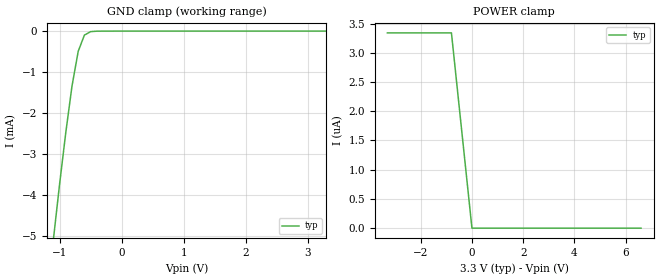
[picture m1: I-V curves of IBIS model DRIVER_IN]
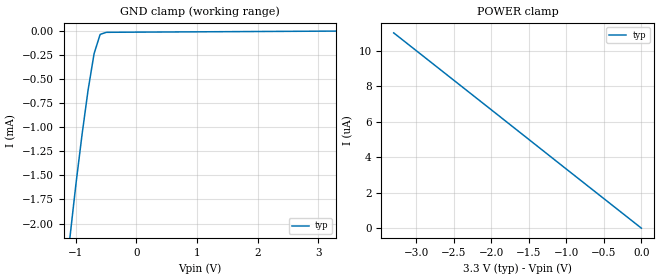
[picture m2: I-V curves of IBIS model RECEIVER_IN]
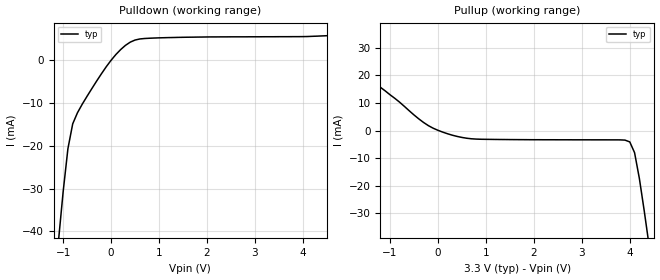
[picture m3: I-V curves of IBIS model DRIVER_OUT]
|   Texas Instruments Incorporated
|   Data Transmissions Products
|   IBIS Model for SN65LVDS179
|   8D SOIC Package
[IBIS Ver]   2.1
[Comment char]   |_char
[File name]   lvds179.ibs
[File Rev]   2.1
[Date]   03/24/2009
[Source]   File originated at Texas Instruments Incorporated.
   Data Transmission Products Group.
[Notes]   Revision History:
   Rev 2.0: 11/05/1998
   - Initial version
   Rev 2.1: 03/24/2009
   - Added Y and Z pins to [Diff pin] list
   - removed warning related to DRIVER_IN powerclamp
[Disclaimer]
(C) Copyright Texas Instruments Incorporated 1998
   All rights reserved
  Texas Instruments Incorporated hereby grants the user of this IBIS
model a non-exclusive, nontransferable license to use this IBIS model
under the following terms.  Before using this IBIS model, the user
should read this license.  If the user does not accept these terms,
the IBIS model should be returned to Texas Instruments within 30 days.
  The user is granted this license only to use the IBIS model and
is not granted rights to sell, load, rent, lease or license the IBIS
model in whole or in part, or in modified form to anyone other than
user.  User may modify the IBIS model to suit its specific applications
but rights to derivative works and such modifications shall belong to
Texas Instruments.
  This IBIS model is provided on an "AS IS" basis and Texas Instruments
makes absolutely no warranty with respect to the information contained
herein.  TEXAS INSTRUMENTS DISCLAIMS AND CUSTOMER WAIVES ALL WARRANTIES,
EXPRESS OR IMPLIED, INCLUDING WARRANTIES OF MERCHANTABILITY OR FITNESS
FOR A PARTICULAR PURPOSE. The entire risk as to quality and performance
is with the Customer. ACCORDINGLY, IN NO EVENT SHALL THE COMPANY BE LIABLE
FOR ANY DAMAGES, WHETHER IN CONTRACT OR TORT,INCLUDING ANY LOST PROFITS
OR OTHER INCIDENTAL, CONSEQUENTIAL, EXEMPLARY, OR PUNITIVE DAMAGES ARISING
OUT OF THE USE OR APPLICATION OF THE IBIS model provided in this package.
Further, Texas Instruments reserves the right to discontinue or make changes
without notice to any product herein to improve reliability, function, or
design. Texas Instruments does not convey any license under patent rights
or any other intellectual property rights, including those of third parties.
Contact Texas Instruments at ATTN:DATA TRANSMISSIONS
Thomas Fisher 8505 Forest Lane, M/S 8710, Dallas, TX 75243-4136
[Copyright]   Copyright 1998, Texas Instruments, All Rights Reserved
[Component]   LVDS179D
[Manufacturer]  Texas Instruments Incorporated
[Package]
|   typ   min   max
R_pkg   0.036   0.033   0.039
L_pkg   3.340nH   2.445nH   4.233nH
C_pkg   0.470pF   0.308pF   0.631pF
[Pin]   signal_name   model_name   R_pin   L_pin   C_pin
1   VCC   POWER   0.034   4.233n   0.630p
2   R   RECEIVER_OUT   0.038   2.445n   0.309p
3   D   DRIVER_IN   0.039   2.448n   0.309p
4   GND   GND   0.033   4.231n   0.631p
5   Y   DRIVER_OUT   0.033   4.230n   0.630p
6   Z   DRIVER_OUT   0.039   2.450n   0.308p
7   B   RECEIVER_IN   0.039   2.448n   0.309p
8   A   RECEIVER_IN   0.033   4.231n   0.630p
[Diff_pin]   inv_pin   vdiff   tdelay_typ   tdelay_min   tdelay_max
| The 'A' pin is Diff_pin and the 'B' pin is the inv_pin
8   7   0.100   0 0 0
5   6   0.300   0 0 0
| Models and submodels in the file (4): DRIVER_IN (Input), RECEIVER_IN (Input), DRIVER_OUT (Output), RECEIVER_OUT (Output)
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|   Driver Input MODEL
[Model]   DRIVER_IN
Model_type   Input
|Signals   D
Vinh = 2.0
Vinl = 0.8
|   typ   min   max
C_comp   1.0pF   NA   NA
|   typ   min   max
[Temperature Range]   25.0   NA   NA
[Voltage range]   3.3V   3.0V   3.6V
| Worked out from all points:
|   GND clamp passes 1 mA (typ) near -0.76 V on its own axis
[GND_clamp]
|   Voltage   I(typ)   I(min)   I(max)
-3.3V     -43.1mA    NA         NA
-1.1V     -5.08mA    NA         NA
-1V       -3.73mA    NA         NA
-900mV    -2.47mA    NA         NA
-800mV    -1.34mA    NA         NA
-700mV    -493uA     NA         NA
-600mV    -98.5uA    NA         NA
-500mV    -13.3uA    NA         NA
3.3V      3.34pA     NA         NA
[Power_clamp]
| Note that the[POWER_clamp]voltage table is referenced to Vcc
| and is calculated using Vtable=Vcc - Vmeasured.
|   Voltage   I(typ)   I(min)   I(max)
-3.3V     3.34uA     NA         NA
-2.7V     3.34uA     NA         NA
-2V       3.34uA     NA         NA
-800mV    3.34uA     NA         NA
0V        0A         NA         NA
6.6V      0A         NA         NA
|   Receiver Input MODEL
[Model]   RECEIVER_IN
Model_type   Input
|Signals   A,B
Vinh = 2.0
Vinl = 0.8
|   typ   min   max
C_comp   1.0pF   NA   NA
|   typ   min   max
[Temperature Range]   25.0   NA   NA
[Voltage range]   3.3V   3.0V   3.6V
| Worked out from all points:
|   GND clamp passes 1 mA (typ) near -0.88 V on its own axis
[GND_clamp]
|   Voltage   I(typ)   I(min)   I(max)
-3.3V     -22.5mA    NA         NA
-1.1V     -2.15mA    NA         NA
-1V       -1.59mA    NA         NA
-900mV    -1.08mA    NA         NA
-800mV    -616uA     NA         NA
-700mV    -234uA     NA         NA
-600mV    -34.5uA    NA         NA
-500mV    -13.2uA    NA         NA
-400mV    -12.3uA    NA         NA
3.3V      444pA      NA         NA
[Power_clamp]
| Note that the[POWER_clamp]voltage table is referenced to Vcc
| and is calculated using Vtable=Vcc - Vmeasured.
|   Voltage   I(typ)   I(min)   I(max)
-3.3V     11uA       NA         NA
-2V       6.67uA     NA         NA
-1V       3.33uA     NA         NA
0V        0A         NA         NA
|   Driver Output  MODEL
[Model]   DRIVER_OUT
Model_type   Output
| Signals   Y,Z
Vmeas = 1.2V   |Reference voltage for timing measurements
Cref = 5pF   |Timing specification test load capacitance value
Rref = 50   |Note: 50 Ohm load; single ended configuration
Vref = 1.18V   |Timing specification test load voltage
| variable   typ   min   max
C_comp   1.0pF   NA   NA
|   typ   min   max
[Temperature Range]   25.0   NA   NA
[Voltage range]   3.3V   3.0V   3.6V
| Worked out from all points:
|   slope of the pulldown table from 0 to 0.495 V, typ, clamps not added: 105 ohm
|   slope of the pullup table from 0 to 0.495 V, typ, clamps not added: 192 ohm
[Pulldown]
|   Voltage   I(typ)   I(min)   I(max)
-3.3V     -348mA     NA         NA
-1.1V     -42.6mA    NA         NA
-1V       -30.8mA    NA         NA
-900mV    -20.7mA    NA         NA
-800mV    -14.9mA    NA         NA
-600mV    -10.3mA    NA         NA
-100mV    -1.58mA    NA         NA
200mV     2.42mA     NA         NA
500mV     4.64mA     NA         NA
1.4V      5.26mA     NA         NA
4.1V      5.46mA     NA         NA
6.6V      7.11mA     NA         NA
[Pullup]
|   Voltage   I(typ)   I(min)   I(max)
| Note that the[Pullup]voltage table is referenced to Vcc
| and is calculated using Vtable=Vcc - Vmeasured.
-3.3V     49.3mA     NA         NA
-2.6V     37.7mA     NA         NA
-1.9V     25.6mA     NA         NA
-400mV    4.24mA     NA         NA
200mV     -1.17mA    NA         NA
800mV     -3.11mA    NA         NA
4V        -4.13mA    NA         NA
4.1V      -8.04mA    NA         NA
4.2V      -17.4mA    NA         NA
4.3V      -29mA      NA         NA
4.4V      -41.4mA    NA         NA
6.6V      -348mA     NA         NA
[Ramp]
|   typ   min   max
dV/dt_r   0.201/800ps   NA   NA
dV/dt_f   0.201/800ps   NA   NA
R_load = 100ohm | Note: The measurement is on a differential configuration
